| IBIS file stm32u595_599_5a5_5a9_lqfp144.ibs
[IBIS ver] 4.2
[File name] stm32u595_599_5a5_5a9_lqfp144.ibs
[File Rev] rev2.0
[Date]  11-09-2023
[Source] Data Created at STMicroelectronics
[Notes]  File originated from ELDO simulations.
[Disclaimer]  This information is for modeling purpose only and is
   not guaranteed. The information is subject to change without
   notice.
[Copyright] Copyright 2023 STMicroelectronics Inc.
|   Component stm32u595_599_5a5_5a9_lqfp144
[Component] stm32u595_599_5a5_5a9_lqfp144
[Manufacturer] STMicroelectronics
[Package]
| variable   typ   min   max
R_pkg  0  NA  NA
L_pkg  0  NA  NA
C_pkg  0  NA  NA
[Pin]   signal_name   model_name
1  PE2  io8_100m_hslv_ft
2  PE3  io8_100m_hslv_tamp_ft
3  PE4  io8_100m_hslv_tamp_ft
4  PE5  io8_100m_hslv_tamp_ft
5  PE6  io8_100m_hslv_tamp_ft
6  VBAT  power
7  PC13  io8_100m_ft
8  PC14-OSC32_IN  nc
9  PC15-OSC32_OUT  nc
10  PF0  io8_100m_hslv_ft
11  PF1  io8_100m_hslv_ft
12  PF2  io8_100m_hslv_ft
13  PF3  io8_100m_hslv_ft
14  PF4  io8_spi_ft
15  PF5  io8_spi_ft
16  VSS  gnd
17  VDD  power
18  PF6  io8_100m_hslv_ft
19  PF7  io8_100m_hslv_ft
20  PF8  io8_100m_hslv_ft
21  PF9  io8_100m_hslv_ft
22  PF10  io8_166m_hslv_ft
23  PH0-OSC_IN  nc
24  PH1-OSC_OUT   nc
25  NRST  nc
26  PC0  io8_100m_hslv_ft
27  PC1  io8_spi_hslv_ft
28  PC2  io8_100m_hslv_ft
29  PC3  io8_100m_hslv_ft
30  VSSA  nc
31  VREFM  nc
32  VREFP  nc
33  VDDA  nc
34  PA0  io8_100m_hslv_tamp_ft
35  PA1  io8_100m_hslv_tamp_ft
36  PA2  io8_100m_hslv_ft
37  PA3  io8_166m_hslv_ft
38  VSS  gnd
39  VDD  power
40  PA4  io8_100m_hslv_ft
41  PA5  io8_100m_ft
42  PA6  io8_100m_hslv_ft
43  PA7  io8_100m_hslv_ft
44  PC4  io8_100m_hslv_ft
45  PC5  io8_100m_tamp_ft
46  PB0  io8_100m_hslv_ft
47  PB1  io8_100m_hslv_ft
48  PB2  io8_100m_hslv_tamp_ft
49  PF11  io8_166m_hslv_ft
50  PF12  io8_100m_hslv_ft
51  VSS  gnd
52  VDD  power
53  PF13  io8_100m_hslv_ft
54  PF14  io8_100m_hslv_ft
55  PF15  io8_100m_hslv_ft
56  PG0  io8_100m_hslv_ft
57  PG1  io8_100m_hslv_ft
58  PE7  io8_100m_hslv_ft
59  PE8  io8_100m_hslv_ft
60  PE9  io8_166m_hslv_ft
61  VSS  gnd
62  VDD  power
63  PE10  io8_166m_hslv_ft
64  PE11  io8_100m_hslv_ft
65  PE12  io8_100m_hslv_ft
66  PE13  io8_100m_hslv_ft
67  PE14  io8_100m_hslv_ft
68  PE15  io8_100m_hslv_ft
69  PB10  io8_spi_hslv_ft
70  VCAP  nc
71  VSSA  nc
72  VDD  power
73  PB12  io8_166m_hslv_ft
74  PB13  io8_100m_i2c_ft
75  PB14  io8_100m_i2c_ft
76  PB15  nc
77  PD8  io8_100m_hslv_ft
78  PD9  io8_100m_hslv_ft
79  PD10  io8_100m_hslv_ft
80  PD11  io8_100m_hslv_ft
81  PD12  io8_100m_hslv_ft
82  PD13  io8_100m_hslv_ft
83  VSS  gnd
84  VDD  power
85  PD14  io8_100m_hslv_ft
86  PD15  io8_100m_hslv_ft
87  PG2  io8_100m_hslv_ft
88  PG3  io8_100m_hslv_ft
89  PG4  io8_100m_hslv_ft
90  PG5  io8_100m_hslv_ft
91  PG6  io8_100m_hslv_ft
92  PG7  io8_100m_hslv_ft
93  PG8  io8_100m_i2c_ft
94  VSS  gnd
95  VDDIO2  power
96  PC6  io8_100m_ft
97  PC7  io8_100m_ft
98  PC8  io8_100m_ft
99  PC9  io8_100m_ft
100  PA8  io8_166m_hslv_ft
101  PA9  io8_100m_usb_vbus_ft
102  PA10  io8_100m_usb_id
103  PA11  io8_100m_ft
104  PA12  io8_100m_ft
105  PA13  io8_100m_ft
106  VDDUSB  power
107  VSS  gnd
108  VDD  power
109  PA14  io8_100m_ft
110  PA15  nc
111  PC10  io8_100m_ft
112  PC11  io8_100m_hslv_ft
113  PC12  io8_166m_hslv_ft
114  PD0  io8_100m_hslv_ft
115  PD1  io8_100m_hslv_ft
116  PD2  io8_100m_ft
117  PD3  io8_166m_hslv_ft
118  PD4  io8_100m_hslv_ft
119  PD5  io8_100m_hslv_ft
120  VSS  gnd
121  VDD  power
122  PD6  io8_166m_hslv_ft
123  PD7  io8_100m_hslv_ft
124  PG9  io8_100m_hslv_ft
125  PG10  io8_100m_hslv_ft
126  PG11  io8_100m_hslv_ft
127  PG12  io8_100m_hslv_ft
128  PG13  io8_100m_hslv_ft
129  PG14  io8_100m_hslv_ft
130  VSS  gnd
131  VDDIO2  power
132  PG15  io8_100m_hslv_ft
133  PB3  io8_100m_i2c_ft
134  PB4  io8_100m_i2c_ft
135  PB5  io8_166m_hslv_ft
136  PB6  io8_100m_i2c_ft
137  PB7  io8_spi_hslv_ft
138  PH3-BOOT0  nc
139  PB8  io8_100m_i2c_ft
140  PB9  io8_100m_i2c_ft
141  PE0  io8_100m_hslv_ft
142  PE1  io8_100m_hslv_ft
143  VSS  gnd
144  VDD  power
[Package Model]   481-lqfp-20x20-144-ldo-230228
[Pin Mapping]   pulldown_ref   pullup_ref   | Comment
1  gndio  vddiom
2  gndio  vddiom
3  gndio  vddiom
4  gndio  vddiom
5  gndio  vddiom
6  nc  vsw
7  gndio  vddiom  | Depending on IO usage
| 7  gndio  vsw  | Depending on IO usage
8  nc  nc
9  nc  nc
10  gndio  vddiom
11  gndio  vddiom
12  gndio  vddiom
13  gndio  vddiom
14  gndio  vddiom
15  gndio  vddiom
16  gndio  nc
17  nc  vddiom
18  gndio  vddiom
19  gndio  vddiom
20  gndio  vddiom
21  gndio  vddiom
22  gndio  vddiom
23  nc  nc
24  nc  nc
25  nc  nc
26  gndio  vddiom
27  gndio  vddiom
28  gndio  vddiom
29  gndio  vddiom
30  nc  nc
31  nc  nc
32  nc  nc
33  nc  nc
34  gndio  vddiom
35  gndio  vddiom
36  gndio  vddiom
37  gndio  vddiom
38  gndio  nc
39  nc  vddiom
40  gndio  vddiom
41  gndio  vddiom
42  gndio  vddiom
43  gndio  vddiom
44  gndio  vddiom
45  gndio  vddiom
46  gndio  vddiom
47  gndio  vddiom
48  gndio  vddiom
49  gndio  vddiom
50  gndio  vddiom
51  gndio  nc
52  nc  vddiom
53  gndio  vddiom
54  gndio  vddiom
55  gndio  vddiom
56  gndio  vddiom
57  gndio  vddiom
58  gndio  vddiom
59  gndio  vddiom
60  gndio  vddiom
61  gndio  nc
62  nc  vddiom
63  gndio  vddiom
64  gndio  vddiom
65  gndio  vddiom
66  gndio  vddiom
67  gndio  vddiom
68  gndio  vddiom
69  gndio  vddiom
70  nc  nc
71  nc  nc
72  nc  vddiom
73  gndio  vddiom
74  gndio  vddiom
75  gndio  vddiom
76  nc  nc
77  gndio  vddiom
78  gndio  vddiom
79  gndio  vddiom
80  gndio  vddiom
81  gndio  vddiom
82  gndio  vddiom
83  gndio  nc
84  nc  vddiom
85  gndio  vddiom
86  gndio  vddiom
87  gndio  vddiom  | Depending on IO usage
| 87  gndio  vddio2  | Depending on IO usage
88  gndio  vddiom  | Depending on IO usage
| 88  gndio  vddio2  | Depending on IO usage
89  gndio  vddiom  | Depending on IO usage
| 89  gndio  vddio2  | Depending on IO usage
90  gndio  vddiom  | Depending on IO usage
| 90  gndio  vddio2  | Depending on IO usage
91  gndio  vddiom  | Depending on IO usage
| 91  gndio  vddio2  | Depending on IO usage
92  gndio  vddiom  | Depending on IO usage
| 92  gndio  vddio2  | Depending on IO usage
93  gndio  vddiom  | Depending on IO usage
| 93  gndio  vddio2  | Depending on IO usage
94  gndio  nc
95  nc  vddio2
96  gndio  vddiom
97  gndio  vddiom
98  gndio  vddiom
99  gndio  vddiom
100  gndio  vddiom
101  gndio  vddiom  | Depending on IO usage
| 101  gndio  vddusb  | Depending on IO usage
102  gndio  vddiom  | Depending on IO usage
| 102  gndio  vddusb  | Depending on IO usage
103  gndio  vddiom  | Depending on IO usage
| 103  gndio  vddusb  | Depending on IO usage
104  gndio  vddiom  | Depending on IO usage
| 104  gndio  vddusb  | Depending on IO usage
105  gndio  vddiom  | Depending on IO usage
| 105  gndio  vddusb  | Depending on IO usage
106  nc  vddusb
107  gndio  nc
108  nc  vddiom
109  gndio  vddiom
110  nc  nc
111  gndio  vddiom
112  gndio  vddiom
113  gndio  vddiom
114  gndio  vddiom
115  gndio  vddiom
116  gndio  vddiom
117  gndio  vddiom
118  gndio  vddiom
119  gndio  vddiom
120  gndio  nc
121  nc  vddiom
122  gndio  vddiom
123  gndio  vddiom
124  gndio  vddiom  | Depending on IO usage
| 124  gndio  vddio2  | Depending on IO usage
125  gndio  vddiom  | Depending on IO usage
| 125  gndio  vddio2  | Depending on IO usage
126  gndio  vddiom  | Depending on IO usage
| 126  gndio  vddio2  | Depending on IO usage
127  gndio  vddiom  | Depending on IO usage
| 127  gndio  vddio2  | Depending on IO usage
128  gndio  vddiom  | Depending on IO usage
| 128  gndio  vddio2  | Depending on IO usage
129  gndio  vddiom  | Depending on IO usage
| 129  gndio  vddio2  | Depending on IO usage
130  gndio  nc
131  nc  vddio2
132  gndio  vddiom  | Depending on IO usage
| 132  gndio  vddio2  | Depending on IO usage
133  gndio  vddiom
134  gndio  vddiom
135  gndio  vddiom
136  gndio  vddiom
137  gndio  vddiom
138  nc  nc
139  gndio  vddiom
140  gndio  vddiom
141  gndio  vddiom
142  gndio  vddiom
143  gndio  nc
144  nc  vddiom
[Model Selector] io8_100m_ft
io8_100m_ft_hs_1v2  "IO8_FT 100MHz high speed @ 1.2V"
io8_100m_ft_fs_1v2  "IO8_FT 100MHz fast speed @ 1.2V"
io8_100m_ft_fs_pd_1v2  "IO8_FT 100MHz fast speed @ 1.2V pulldown"
io8_100m_ft_ms_1v2  "IO8_FT 100MHz med speed @ 1.2V"
io8_100m_ft_ms_pd_1v2  "IO8_FT 100MHz med speed @ 1.2V pulldown"
io8_100m_ft_ls_1v2  "IO8_FT 100MHz low speed @ 1.2V"
io8_100m_ft_ls_pd_1v2  "IO8_FT 100MHz low speed @ 1.2V pulldown"
io8_100m_ft_hs_1v8  "IO8_FT 100MHz high speed @ 1.8V"
io8_100m_ft_hs_pd_1v8  "IO8_FT 100MHz high speed @ 1.8V pulldown"
io8_100m_ft_fs_1v8  "IO8_FT 100MHz fast speed @ 1.8V"
io8_100m_ft_fs_pd_1v8  "IO8_FT 100MHz fast speed @ 1.8V pulldown"
io8_100m_ft_ms_1v8  "IO8_FT 100MHz med speed @ 1.8V"
io8_100m_ft_ms_pd_1v8  "IO8_FT 100MHz med speed @ 1.8V pulldown"
io8_100m_ft_ls_1v8  "IO8_FT 100MHz low speed @ 1.8V"
io8_100m_ft_ls_pd_1v8  "IO8_FT 100MHz low speed @ 1.8V pulldown"
io8_100m_ft_hs_3v3  "IO8_FT 100MHz high speed @ 3.3V"
io8_100m_ft_hs_pd_3v3  "IO8_FT 100MHz high speed @ 3.3V pulldown"
io8_100m_ft_fs_3v3  "IO8_FT 100MHz fast speed @ 3.3V"
io8_100m_ft_fs_pd_3v3  "IO8_FT 100MHz fast speed @ 3.3V pulldown"
io8_100m_ft_ms_3v3  "IO8_FT 100MHz med speed @ 3.3V"
io8_100m_ft_ms_pd_3v3  "IO8_FT 100MHz med speed @ 3.3V pulldown"
io8_100m_ft_ls_3v3  "IO8_FT 100MHz low speed @ 3.3V"
io8_100m_ft_ls_pd_3v3  "IO8_FT 100MHz low speed @ 3.3V pulldown"
[Model Selector] io8_100m_hslv_ft
io8_100m_ft_hs_1v2  "IO8_FT 100MHz high speed @ 1.2V"
io8_100m_ft_hs_pu_1v2  "IO8_FT 100MHz high speed @ 1.2V pullup"
io8_100m_ft_hs_pd_1v2  "IO8_FT 100MHz high speed @ 1.2V pulldown"
io8_100m_ft_fs_1v2  "IO8_FT 100MHz fast speed @ 1.2V"
io8_100m_ft_fs_pu_1v2  "IO8_FT 100MHz fast speed @ 1.2V pullup"
io8_100m_ft_fs_pd_1v2  "IO8_FT 100MHz fast speed @ 1.2V pulldown"
io8_100m_ft_ms_1v2  "IO8_FT 100MHz med speed @ 1.2V"
io8_100m_ft_ms_pu_1v2  "IO8_FT 100MHz med speed @ 1.2V pullup"
io8_100m_ft_ms_pd_1v2  "IO8_FT 100MHz med speed @ 1.2V pulldown"
io8_100m_ft_ls_1v2  "IO8_FT 100MHz low speed @ 1.2V"
io8_100m_ft_ls_pu_1v2  "IO8_FT 100MHz low speed @ 1.2V pullup"
io8_100m_ft_ls_pd_1v2  "IO8_FT 100MHz low speed @ 1.2V pulldown"
io8_100m_ft_hs_1v8  "IO8_FT 100MHz high speed @ 1.8V"
io8_100m_ft_hs_pu_1v8  "IO8_FT 100MHz high speed @ 1.8V pullup"
io8_100m_ft_hs_pd_1v8  "IO8_FT 100MHz high speed @ 1.8V pulldown"
io8_100m_ft_fs_1v8  "IO8_FT 100MHz fast speed @ 1.8V"
io8_100m_ft_fs_pu_1v8  "IO8_FT 100MHz fast speed @ 1.8V pullup"
io8_100m_ft_fs_pd_1v8  "IO8_FT 100MHz fast speed @ 1.8V pulldown"
io8_100m_ft_ms_1v8  "IO8_FT 100MHz med speed @ 1.8V"
io8_100m_ft_ms_pu_1v8  "IO8_FT 100MHz med speed @ 1.8V pullup"
io8_100m_ft_ms_pd_1v8  "IO8_FT 100MHz med speed @ 1.8V pulldown"
io8_100m_ft_ls_1v8  "IO8_FT 100MHz low speed @ 1.8V"
io8_100m_ft_ls_pu_1v8  "IO8_FT 100MHz low speed @ 1.8V pullup"
io8_100m_ft_ls_pd_1v8  "IO8_FT 100MHz low speed @ 1.8V pulldown"
io8_100m_ft_hs_3v3  "IO8_FT 100MHz high speed @ 3.3V"
io8_100m_ft_hs_pu_3v3  "IO8_FT 100MHz high speed @ 3.3V pullup"
io8_100m_ft_hs_pd_3v3  "IO8_FT 100MHz high speed @ 3.3V pulldown"
io8_100m_ft_fs_3v3  "IO8_FT 100MHz fast speed @ 3.3V"
io8_100m_ft_fs_pu_3v3  "IO8_FT 100MHz fast speed @ 3.3V pullup"
io8_100m_ft_fs_pd_3v3  "IO8_FT 100MHz fast speed @ 3.3V pulldown"
io8_100m_ft_ms_3v3  "IO8_FT 100MHz med speed @ 3.3V"
io8_100m_ft_ms_pu_3v3  "IO8_FT 100MHz med speed @ 3.3V pullup"
io8_100m_ft_ms_pd_3v3  "IO8_FT 100MHz med speed @ 3.3V pulldown"
io8_100m_ft_ls_3v3  "IO8_FT 100MHz low speed @ 3.3V"
io8_100m_ft_ls_pu_3v3  "IO8_FT 100MHz low speed @ 3.3V pullup"
io8_100m_ft_ls_pd_3v3  "IO8_FT 100MHz low speed @ 3.3V pulldown"
io8_100m_hslv_ft_hs_1v2  "IO8_FT 100MHz HSLV high speed @ 1.2V"
io8_100m_hslv_ft_hs_pu_1v2  "IO8_FT 100MHz HSLV high speed @ 1.2V pullup"
io8_100m_hslv_ft_hs_pd_1v2  "IO8_FT 100MHz HSLV high speed @ 1.2V pulldown"
io8_100m_hslv_ft_fs_1v2  "IO8_FT 100MHz HSLV fast speed @ 1.2V"
io8_100m_hslv_ft_fs_pu_1v2  "IO8_FT 100MHz HSLV fast speed @ 1.2V pullup"
io8_100m_hslv_ft_fs_pd_1v2  "IO8_FT 100MHz HSLV fast speed @ 1.2V pulldown"
io8_100m_hslv_ft_ms_1v2  "IO8_FT 100MHz HSLV med speed @ 1.2V"
io8_100m_hslv_ft_ms_pu_1v2  "IO8_FT 100MHz HSLV med speed @ 1.2V pullup"
io8_100m_hslv_ft_ms_pd_1v2  "IO8_FT 100MHz HSLV med speed @ 1.2V pulldown"
io8_100m_hslv_ft_ls_1v2  "IO8_FT 100MHz HSLV low speed @ 1.2V"
io8_100m_hslv_ft_ls_pu_1v2  "IO8_FT 100MHz HSLV low speed @ 1.2V pullup"
io8_100m_hslv_ft_ls_pd_1v2  "IO8_FT 100MHz HSLV low speed @ 1.2V pulldown"
io8_100m_hslv_ft_hs_1v8  "IO8_FT 100MHz HSLV high speed @ 1.8V"
io8_100m_hslv_ft_hs_pu_1v8  "IO8_FT 100MHz HSLV high speed @ 1.8V pullup"
io8_100m_hslv_ft_hs_pd_1v8  "IO8_FT 100MHz HSLV high speed @ 1.8V pulldown"
io8_100m_hslv_ft_fs_1v8  "IO8_FT 100MHz HSLV fast speed @ 1.8V"
io8_100m_hslv_ft_fs_pu_1v8  "IO8_FT 100MHz HSLV fast speed @ 1.8V pullup"
io8_100m_hslv_ft_fs_pd_1v8  "IO8_FT 100MHz HSLV fast speed @ 1.8V pulldown"
io8_100m_hslv_ft_ms_1v8  "IO8_FT 100MHz HSLV med speed @ 1.8V"
io8_100m_hslv_ft_ms_pu_1v8  "IO8_FT 100MHz HSLV med speed @ 1.8V pullup"
io8_100m_hslv_ft_ms_pd_1v8  "IO8_FT 100MHz HSLV med speed @ 1.8V pulldown"
io8_100m_hslv_ft_ls_1v8  "IO8_FT 100MHz HSLV low speed @ 1.8V"
io8_100m_hslv_ft_ls_pu_1v8  "IO8_FT 100MHz HSLV low speed @ 1.8V pullup"
io8_100m_hslv_ft_ls_pd_1v8  "IO8_FT 100MHz HSLV low speed @ 1.8V pulldown"
io8_100m_hslv_ft_hs_2v5  "IO8_FT 100MHz HSLV high speed @ 2.5V"
io8_100m_hslv_ft_hs_pu_2v5  "IO8_FT 100MHz HSLV high speed @ 2.5V pullup"
io8_100m_hslv_ft_hs_pd_2v5  "IO8_FT 100MHz HSLV high speed @ 2.5V pulldown"
io8_100m_hslv_ft_fs_2v5  "IO8_FT 100MHz HSLV fast speed @ 2.5V"
io8_100m_hslv_ft_fs_pu_2v5  "IO8_FT 100MHz HSLV fast speed @ 2.5V pullup"
io8_100m_hslv_ft_fs_pd_2v5  "IO8_FT 100MHz HSLV fast speed @ 2.5V pulldown"
io8_100m_hslv_ft_ms_2v5  "IO8_FT 100MHz HSLV med speed @ 2.5V"
io8_100m_hslv_ft_ms_pu_2v5  "IO8_FT 100MHz HSLV med speed @ 2.5V pullup"
io8_100m_hslv_ft_ms_pd_2v5  "IO8_FT 100MHz HSLV med speed @ 2.5V pulldown"
io8_100m_hslv_ft_ls_2v5  "IO8_FT 100MHz HSLV low speed @ 2.5V"
io8_100m_hslv_ft_ls_pu_2v5  "IO8_FT 100MHz HSLV low speed @ 2.5V pullup"
io8_100m_hslv_ft_ls_pd_2v5  "IO8_FT 100MHz HSLV low speed @ 2.5V pulldown"
[Model Selector] io8_100m_hslv_tamp_ft
io8_100m_ft_hs_1v2  "IO8_FT 100MHz high speed @ 1.2V"
io8_100m_ft_hs_pu_1v2  "IO8_FT 100MHz high speed @ 1.2V pullup"
io8_100m_ft_hs_pd_1v2  "IO8_FT 100MHz high speed @ 1.2V pulldown"
io8_100m_ft_fs_1v2  "IO8_FT 100MHz fast speed @ 1.2V"
io8_100m_ft_fs_pu_1v2  "IO8_FT 100MHz fast speed @ 1.2V pullup"
io8_100m_ft_fs_pd_1v2  "IO8_FT 100MHz fast speed @ 1.2V pulldown"
io8_100m_ft_ms_1v2  "IO8_FT 100MHz med speed @ 1.2V"
io8_100m_ft_ms_pu_1v2  "IO8_FT 100MHz med speed @ 1.2V pullup"
io8_100m_ft_ms_pd_1v2  "IO8_FT 100MHz med speed @ 1.2V pulldown"
io8_100m_ft_ls_1v2  "IO8_FT 100MHz low speed @ 1.2V"
io8_100m_ft_ls_pu_1v2  "IO8_FT 100MHz low speed @ 1.2V pullup"
io8_100m_ft_ls_pd_1v2  "IO8_FT 100MHz low speed @ 1.2V pulldown"
io8_100m_ft_hs_1v8  "IO8_FT 100MHz high speed @ 1.8V"
io8_100m_ft_hs_pu_1v8  "IO8_FT 100MHz high speed @ 1.8V pullup"
io8_100m_ft_hs_pd_1v8  "IO8_FT 100MHz high speed @ 1.8V pulldown"
io8_100m_ft_fs_1v8  "IO8_FT 100MHz fast speed @ 1.8V"
io8_100m_ft_fs_pu_1v8  "IO8_FT 100MHz fast speed @ 1.8V pullup"
io8_100m_ft_fs_pd_1v8  "IO8_FT 100MHz fast speed @ 1.8V pulldown"
io8_100m_ft_ms_1v8  "IO8_FT 100MHz med speed @ 1.8V"
io8_100m_ft_ms_pu_1v8  "IO8_FT 100MHz med speed @ 1.8V pullup"
io8_100m_ft_ms_pd_1v8  "IO8_FT 100MHz med speed @ 1.8V pulldown"
io8_100m_ft_ls_1v8  "IO8_FT 100MHz low speed @ 1.8V"
io8_100m_ft_ls_pu_1v8  "IO8_FT 100MHz low speed @ 1.8V pullup"
io8_100m_ft_ls_pd_1v8  "IO8_FT 100MHz low speed @ 1.8V pulldown"
io8_100m_ft_hs_3v3  "IO8_FT 100MHz high speed @ 3.3V"
io8_100m_ft_hs_pu_3v3  "IO8_FT 100MHz high speed @ 3.3V pullup"
io8_100m_ft_hs_pd_3v3  "IO8_FT 100MHz high speed @ 3.3V pulldown"
io8_100m_ft_fs_3v3  "IO8_FT 100MHz fast speed @ 3.3V"
io8_100m_ft_fs_pu_3v3  "IO8_FT 100MHz fast speed @ 3.3V pullup"
io8_100m_ft_fs_pd_3v3  "IO8_FT 100MHz fast speed @ 3.3V pulldown"
io8_100m_ft_ms_3v3  "IO8_FT 100MHz med speed @ 3.3V"
io8_100m_ft_ms_pu_3v3  "IO8_FT 100MHz med speed @ 3.3V pullup"
io8_100m_ft_ms_pd_3v3  "IO8_FT 100MHz med speed @ 3.3V pulldown"
io8_100m_ft_ls_3v3  "IO8_FT 100MHz low speed @ 3.3V"
io8_100m_ft_ls_pu_3v3  "IO8_FT 100MHz low speed @ 3.3V pullup"
io8_100m_ft_ls_pd_3v3  "IO8_FT 100MHz low speed @ 3.3V pulldown"
io8_100m_hslv_ft_hs_1v2  "IO8_FT 100MHz HSLV high speed @ 1.2V"
io8_100m_hslv_ft_hs_pu_1v2  "IO8_FT 100MHz HSLV high speed @ 1.2V pullup"
io8_100m_hslv_ft_hs_pd_1v2  "IO8_FT 100MHz HSLV high speed @ 1.2V pulldown"
io8_100m_hslv_ft_fs_1v2  "IO8_FT 100MHz HSLV fast speed @ 1.2V"
io8_100m_hslv_ft_fs_pu_1v2  "IO8_FT 100MHz HSLV fast speed @ 1.2V pullup"
io8_100m_hslv_ft_fs_pd_1v2  "IO8_FT 100MHz HSLV fast speed @ 1.2V pulldown"
io8_100m_hslv_ft_ms_1v2  "IO8_FT 100MHz HSLV med speed @ 1.2V"
io8_100m_hslv_ft_ms_pu_1v2  "IO8_FT 100MHz HSLV med speed @ 1.2V pullup"
io8_100m_hslv_ft_ms_pd_1v2  "IO8_FT 100MHz HSLV med speed @ 1.2V pulldown"
io8_100m_hslv_ft_ls_1v2  "IO8_FT 100MHz HSLV low speed @ 1.2V"
io8_100m_hslv_ft_ls_pu_1v2  "IO8_FT 100MHz HSLV low speed @ 1.2V pullup"
io8_100m_hslv_ft_ls_pd_1v2  "IO8_FT 100MHz HSLV low speed @ 1.2V pulldown"
io8_100m_hslv_ft_hs_1v8  "IO8_FT 100MHz HSLV high speed @ 1.8V"
io8_100m_hslv_ft_hs_pu_1v8  "IO8_FT 100MHz HSLV high speed @ 1.8V pullup"
io8_100m_hslv_ft_hs_pd_1v8  "IO8_FT 100MHz HSLV high speed @ 1.8V pulldown"
io8_100m_hslv_ft_fs_1v8  "IO8_FT 100MHz HSLV fast speed @ 1.8V"
io8_100m_hslv_ft_fs_pu_1v8  "IO8_FT 100MHz HSLV fast speed @ 1.8V pullup"
io8_100m_hslv_ft_fs_pd_1v8  "IO8_FT 100MHz HSLV fast speed @ 1.8V pulldown"
io8_100m_hslv_ft_ms_1v8  "IO8_FT 100MHz HSLV med speed @ 1.8V"
io8_100m_hslv_ft_ms_pu_1v8  "IO8_FT 100MHz HSLV med speed @ 1.8V pullup"
io8_100m_hslv_ft_ms_pd_1v8  "IO8_FT 100MHz HSLV med speed @ 1.8V pulldown"
io8_100m_hslv_ft_ls_1v8  "IO8_FT 100MHz HSLV low speed @ 1.8V"
io8_100m_hslv_ft_ls_pu_1v8  "IO8_FT 100MHz HSLV low speed @ 1.8V pullup"
io8_100m_hslv_ft_ls_pd_1v8  "IO8_FT 100MHz HSLV low speed @ 1.8V pulldown"
io8_100m_hslv_ft_hs_2v5  "IO8_FT 100MHz HSLV high speed @ 2.5V"
io8_100m_hslv_ft_hs_pu_2v5  "IO8_FT 100MHz HSLV high speed @ 2.5V pullup"
io8_100m_hslv_ft_hs_pd_2v5  "IO8_FT 100MHz HSLV high speed @ 2.5V pulldown"
io8_100m_hslv_ft_fs_2v5  "IO8_FT 100MHz HSLV fast speed @ 2.5V"
io8_100m_hslv_ft_fs_pu_2v5  "IO8_FT 100MHz HSLV fast speed @ 2.5V pullup"
io8_100m_hslv_ft_fs_pd_2v5  "IO8_FT 100MHz HSLV fast speed @ 2.5V pulldown"
io8_100m_hslv_ft_ms_2v5  "IO8_FT 100MHz HSLV med speed @ 2.5V"
io8_100m_hslv_ft_ms_pu_2v5  "IO8_FT 100MHz HSLV med speed @ 2.5V pullup"
io8_100m_hslv_ft_ms_pd_2v5  "IO8_FT 100MHz HSLV med speed @ 2.5V pulldown"
io8_100m_hslv_ft_ls_2v5  "IO8_FT 100MHz HSLV low speed @ 2.5V"
io8_100m_hslv_ft_ls_pu_2v5  "IO8_FT 100MHz HSLV low speed @ 2.5V pullup"
io8_100m_hslv_ft_ls_pd_2v5  "IO8_FT 100MHz HSLV low speed @ 2.5V pulldown"
io8_ft_v33_hs_1v2  "IO8_FT_V33 high speed @ 1.2V"
io8_ft_v33_hs_pu_1v2  "IO8_FT_V33 high speed @ 1.2V pullup"
io8_ft_v33_hs_pd_1v2  "IO8_FT_V33 high speed @ 1.2V pulldown"
io8_ft_v33_fs_1v2  "IO8_FT_V33 fast speed @ 1.2V"
io8_ft_v33_fs_pu_1v2  "IO8_FT_V33 fast speed @ 1.2V pullup"
io8_ft_v33_fs_pd_1v2  "IO8_FT_V33 fast speed @ 1.2V pulldown"
io8_ft_v33_ms_1v2  "IO8_FT_V33 med speed @ 1.2V"
io8_ft_v33_ms_pu_1v2  "IO8_FT_V33 med speed @ 1.2V pullup"
io8_ft_v33_ms_pd_1v2  "IO8_FT_V33 med speed @ 1.2V pulldown"
io8_ft_v33_ls_1v2  "IO8_FT_V33 low speed @ 1.2V"
io8_ft_v33_ls_pu_1v2  "IO8_FT_V33 low speed @ 1.2V pullup"
io8_ft_v33_ls_pd_1v2  "IO8_FT_V33 low speed @ 1.2V pulldown"
io8_ft_v33_hs_1v8  "IO8_FT_V33 high speed @ 1.8V"
io8_ft_v33_hs_pu_1v8  "IO8_FT_V33 high speed @ 1.8V pullup"
io8_ft_v33_hs_pd_1v8  "IO8_FT_V33 high speed @ 1.8V pulldown"
io8_ft_v33_fs_1v8  "IO8_FT_V33 fast speed @ 1.8V"
io8_ft_v33_fs_pu_1v8  "IO8_FT_V33 fast speed @ 1.8V pullup"
io8_ft_v33_fs_pd_1v8  "IO8_FT_V33 fast speed @ 1.8V pulldown"
io8_ft_v33_ms_1v8  "IO8_FT_V33 med speed @ 1.8V"
io8_ft_v33_ms_pu_1v8  "IO8_FT_V33 med speed @ 1.8V pullup"
io8_ft_v33_ms_pd_1v8  "IO8_FT_V33 med speed @ 1.8V pulldown"
io8_ft_v33_ls_1v8  "IO8_FT_V33 low speed @ 1.8V"
io8_ft_v33_ls_pu_1v8  "IO8_FT_V33 low speed @ 1.8V pullup"
io8_ft_v33_ls_pd_1v8  "IO8_FT_V33 low speed @ 1.8V pulldown"
io8_ft_v33_hs_3v3  "IO8_FT_V33 high speed @ 3.3V"
io8_ft_v33_hs_pu_3v3  "IO8_FT_V33 high speed @ 3.3V pullup"
io8_ft_v33_hs_pd_3v3  "IO8_FT_V33 high speed @ 3.3V pulldown"
io8_ft_v33_fs_3v3  "IO8_FT_V33 fast speed @ 3.3V"
io8_ft_v33_fs_pu_3v3  "IO8_FT_V33 fast speed @ 3.3V pullup"
io8_ft_v33_fs_pd_3v3  "IO8_FT_V33 fast speed @ 3.3V pulldown"
io8_ft_v33_ms_3v3  "IO8_FT_V33 med speed @ 3.3V"
io8_ft_v33_ms_pu_3v3  "IO8_FT_V33 med speed @ 3.3V pullup"
io8_ft_v33_ms_pd_3v3  "IO8_FT_V33 med speed @ 3.3V pulldown"
io8_ft_v33_ls_3v3  "IO8_FT_V33 low speed @ 3.3V"
io8_ft_v33_ls_pu_3v3  "IO8_FT_V33 low speed @ 3.3V pullup"
io8_ft_v33_ls_pd_3v3  "IO8_FT_V33 low speed @ 3.3V pulldown"
[Model Selector] io8_100m_i2c_ft
io8_100m_ft_hs_1v2  "IO8_FT 100MHz high speed @ 1.2V"
io8_100m_ft_hs_pu_1v2  "IO8_FT 100MHz high speed @ 1.2V pullup"
io8_100m_ft_hs_pd_1v2  "IO8_FT 100MHz high speed @ 1.2V pulldown"
io8_100m_ft_fs_1v2  "IO8_FT 100MHz fast speed @ 1.2V"
io8_100m_ft_fs_pu_1v2  "IO8_FT 100MHz fast speed @ 1.2V pullup"
io8_100m_ft_fs_pd_1v2  "IO8_FT 100MHz fast speed @ 1.2V pulldown"
io8_100m_ft_ms_1v2  "IO8_FT 100MHz med speed @ 1.2V"
io8_100m_ft_ms_pu_1v2  "IO8_FT 100MHz med speed @ 1.2V pullup"
io8_100m_ft_ms_pd_1v2  "IO8_FT 100MHz med speed @ 1.2V pulldown"
io8_100m_ft_ls_1v2  "IO8_FT 100MHz low speed @ 1.2V"
io8_100m_ft_ls_pu_1v2  "IO8_FT 100MHz low speed @ 1.2V pullup"
io8_100m_ft_ls_pd_1v2  "IO8_FT 100MHz low speed @ 1.2V pulldown"
io8_100m_ft_hs_1v8  "IO8_FT 100MHz high speed @ 1.8V"
io8_100m_ft_hs_pu_1v8  "IO8_FT 100MHz high speed @ 1.8V pullup"
io8_100m_ft_hs_pd_1v8  "IO8_FT 100MHz high speed @ 1.8V pulldown"
io8_100m_ft_fs_1v8  "IO8_FT 100MHz fast speed @ 1.8V"
io8_100m_ft_fs_pu_1v8  "IO8_FT 100MHz fast speed @ 1.8V pullup"
io8_100m_ft_fs_pd_1v8  "IO8_FT 100MHz fast speed @ 1.8V pulldown"
io8_100m_ft_ms_1v8  "IO8_FT 100MHz med speed @ 1.8V"
io8_100m_ft_ms_pu_1v8  "IO8_FT 100MHz med speed @ 1.8V pullup"
io8_100m_ft_ms_pd_1v8  "IO8_FT 100MHz med speed @ 1.8V pulldown"
io8_100m_ft_ls_1v8  "IO8_FT 100MHz low speed @ 1.8V"
io8_100m_ft_ls_pu_1v8  "IO8_FT 100MHz low speed @ 1.8V pullup"
io8_100m_ft_ls_pd_1v8  "IO8_FT 100MHz low speed @ 1.8V pulldown"
io8_100m_ft_hs_3v3  "IO8_FT 100MHz high speed @ 3.3V"
io8_100m_ft_hs_pu_3v3  "IO8_FT 100MHz high speed @ 3.3V pullup"
io8_100m_ft_hs_pd_3v3  "IO8_FT 100MHz high speed @ 3.3V pulldown"
io8_100m_ft_fs_3v3  "IO8_FT 100MHz fast speed @ 3.3V"
io8_100m_ft_fs_pu_3v3  "IO8_FT 100MHz fast speed @ 3.3V pullup"
io8_100m_ft_fs_pd_3v3  "IO8_FT 100MHz fast speed @ 3.3V pulldown"
io8_100m_ft_ms_3v3  "IO8_FT 100MHz med speed @ 3.3V"
io8_100m_ft_ms_pu_3v3  "IO8_FT 100MHz med speed @ 3.3V pullup"
io8_100m_ft_ms_pd_3v3  "IO8_FT 100MHz med speed @ 3.3V pulldown"
io8_100m_ft_ls_3v3  "IO8_FT 100MHz low speed @ 3.3V"
io8_100m_ft_ls_pu_3v3  "IO8_FT 100MHz low speed @ 3.3V pullup"
io8_100m_ft_ls_pd_3v3  "IO8_FT 100MHz low speed @ 3.3V pulldown"
io8_100m_i2c_ft_1v2  "IO8_FT 100MHz I2C @ 1.2V"
io8_100m_i2c_ft_pu_1v2  "IO8_FT 100MHz I2C @ 1.2V pullup"
io8_100m_i2c_ft_pd_1v2  "IO8_FT 100MHz I2C @ 1.2V pulldown"
io8_100m_i2c_ft_1v8  "IO8_FT 100MHz I2C @ 1.8V"
io8_100m_i2c_ft_pu_1v8  "IO8_FT 100MHz I2C @ 1.8V pullup"
io8_100m_i2c_ft_pd_1v8  "IO8_FT 100MHz I2C @ 1,8V pulldown"
io8_100m_i2c_ft_3v3  "IO8_FT 100MHz I2C @ 3.3V"
io8_100m_i2c_ft_pu_3v3  "IO8_FT 100MHz I2C HSLV @ 3.3V pullup"
io8_100m_i2c_ft_pd_3v3  "IO8_FT 100MHz I2C @ 3.3V pulldown"
[Model Selector] io8_100m_tamp_ft
io8_100m_ft_hs_1v2  "IO8_FT 100MHz high speed @ 1.2V"
io8_100m_ft_hs_pu_1v2  "IO8_FT 100MHz high speed @ 1.2V pullup"
io8_100m_ft_hs_pd_1v2  "IO8_FT 100MHz high speed @ 1.2V pulldown"
io8_100m_ft_fs_1v2  "IO8_FT 100MHz fast speed @ 1.2V"
io8_100m_ft_fs_pu_1v2  "IO8_FT 100MHz fast speed @ 1.2V pullup"
io8_100m_ft_fs_pd_1v2  "IO8_FT 100MHz fast speed @ 1.2V pulldown"
io8_100m_ft_ms_1v2  "IO8_FT 100MHz med speed @ 1.2V"
io8_100m_ft_ms_pu_1v2  "IO8_FT 100MHz med speed @ 1.2V pullup"
io8_100m_ft_ms_pd_1v2  "IO8_FT 100MHz med speed @ 1.2V pulldown"
io8_100m_ft_ls_1v2  "IO8_FT 100MHz low speed @ 1.2V"
io8_100m_ft_ls_pu_1v2  "IO8_FT 100MHz low speed @ 1.2V pullup"
io8_100m_ft_ls_pd_1v2  "IO8_FT 100MHz low speed @ 1.2V pulldown"
io8_100m_ft_hs_1v8  "IO8_FT 100MHz high speed @ 1.8V"
io8_100m_ft_hs_pu_1v8  "IO8_FT 100MHz high speed @ 1.8V pullup"
io8_100m_ft_hs_pd_1v8  "IO8_FT 100MHz high speed @ 1.8V pulldown"
io8_100m_ft_fs_1v8  "IO8_FT 100MHz fast speed @ 1.8V"
io8_100m_ft_fs_pu_1v8  "IO8_FT 100MHz fast speed @ 1.8V pullup"
io8_100m_ft_fs_pd_1v8  "IO8_FT 100MHz fast speed @ 1.8V pulldown"
io8_100m_ft_ms_1v8  "IO8_FT 100MHz med speed @ 1.8V"
io8_100m_ft_ms_pu_1v8  "IO8_FT 100MHz med speed @ 1.8V pullup"
io8_100m_ft_ms_pd_1v8  "IO8_FT 100MHz med speed @ 1.8V pulldown"
io8_100m_ft_ls_1v8  "IO8_FT 100MHz low speed @ 1.8V"
io8_100m_ft_ls_pu_1v8  "IO8_FT 100MHz low speed @ 1.8V pullup"
io8_100m_ft_ls_pd_1v8  "IO8_FT 100MHz low speed @ 1.8V pulldown"
io8_100m_ft_hs_3v3  "IO8_FT 100MHz high speed @ 3.3V"
io8_100m_ft_hs_pu_3v3  "IO8_FT 100MHz high speed @ 3.3V pullup"
io8_100m_ft_hs_pd_3v3  "IO8_FT 100MHz high speed @ 3.3V pulldown"
io8_100m_ft_fs_3v3  "IO8_FT 100MHz fast speed @ 3.3V"
io8_100m_ft_fs_pu_3v3  "IO8_FT 100MHz fast speed @ 3.3V pullup"
io8_100m_ft_fs_pd_3v3  "IO8_FT 100MHz fast speed @ 3.3V pulldown"
io8_100m_ft_ms_3v3  "IO8_FT 100MHz med speed @ 3.3V"
io8_100m_ft_ms_pu_3v3  "IO8_FT 100MHz med speed @ 3.3V pullup"
io8_100m_ft_ms_pd_3v3  "IO8_FT 100MHz med speed @ 3.3V pulldown"
io8_100m_ft_ls_3v3  "IO8_FT 100MHz low speed @ 3.3V"
io8_100m_ft_ls_pu_3v3  "IO8_FT 100MHz low speed @ 3.3V pullup"
io8_100m_ft_ls_pd_3v3  "IO8_FT 100MHz low speed @ 3.3V pulldown"
io8_ft_v33_hs_1v2  "IO8_FT_V33 high speed @ 1.2V"
io8_ft_v33_hs_pu_1v2  "IO8_FT_V33 high speed @ 1.2V pullup"
io8_ft_v33_hs_pd_1v2  "IO8_FT_V33 high speed @ 1.2V pulldown"
io8_ft_v33_fs_1v2  "IO8_FT_V33 fast speed @ 1.2V"
io8_ft_v33_fs_pu_1v2  "IO8_FT_V33 fast speed @ 1.2V pullup"
io8_ft_v33_fs_pd_1v2  "IO8_FT_V33 fast speed @ 1.2V pulldown"
io8_ft_v33_ms_1v2  "IO8_FT_V33 med speed @ 1.2V"
io8_ft_v33_ms_pu_1v2  "IO8_FT_V33 med speed @ 1.2V pullup"
io8_ft_v33_ms_pd_1v2  "IO8_FT_V33 med speed @ 1.2V pulldown"
io8_ft_v33_ls_1v2  "IO8_FT_V33 low speed @ 1.2V"
io8_ft_v33_ls_pu_1v2  "IO8_FT_V33 low speed @ 1.2V pullup"
io8_ft_v33_ls_pd_1v2  "IO8_FT_V33 low speed @ 1.2V pulldown"
io8_ft_v33_hs_1v8  "IO8_FT_V33 high speed @ 1.8V"
io8_ft_v33_hs_pu_1v8  "IO8_FT_V33 high speed @ 1.8V pullup"
io8_ft_v33_hs_pd_1v8  "IO8_FT_V33 high speed @ 1.8V pulldown"
io8_ft_v33_fs_1v8  "IO8_FT_V33 fast speed @ 1.8V"
io8_ft_v33_fs_pu_1v8  "IO8_FT_V33 fast speed @ 1.8V pullup"
io8_ft_v33_fs_pd_1v8  "IO8_FT_V33 fast speed @ 1.8V pulldown"
io8_ft_v33_ms_1v8  "IO8_FT_V33 med speed @ 1.8V"
io8_ft_v33_ms_pu_1v8  "IO8_FT_V33 med speed @ 1.8V pullup"
io8_ft_v33_ms_pd_1v8  "IO8_FT_V33 med speed @ 1.8V pulldown"
io8_ft_v33_ls_1v8  "IO8_FT_V33 low speed @ 1.8V"
io8_ft_v33_ls_pu_1v8  "IO8_FT_V33 low speed @ 1.8V pullup"
io8_ft_v33_ls_pd_1v8  "IO8_FT_V33 low speed @ 1.8V pulldown"
io8_ft_v33_hs_3v3  "IO8_FT_V33 high speed @ 3.3V"
io8_ft_v33_hs_pu_3v3  "IO8_FT_V33 high speed @ 3.3V pullup"
io8_ft_v33_hs_pd_3v3  "IO8_FT_V33 high speed @ 3.3V pulldown"
io8_ft_v33_fs_3v3  "IO8_FT_V33 fast speed @ 3.3V"
io8_ft_v33_fs_pu_3v3  "IO8_FT_V33 fast speed @ 3.3V pullup"
io8_ft_v33_fs_pd_3v3  "IO8_FT_V33 fast speed @ 3.3V pulldown"
io8_ft_v33_ms_3v3  "IO8_FT_V33 med speed @ 3.3V"
io8_ft_v33_ms_pu_3v3  "IO8_FT_V33 med speed @ 3.3V pullup"
io8_ft_v33_ms_pd_3v3  "IO8_FT_V33 med speed @ 3.3V pulldown"
io8_ft_v33_ls_3v3  "IO8_FT_V33 low speed @ 3.3V"
io8_ft_v33_ls_pu_3v3  "IO8_FT_V33 low speed @ 3.3V pullup"
io8_ft_v33_ls_pd_3v3  "IO8_FT_V33 low speed @ 3.3V pulldown"
[Model Selector] io8_100m_usb_id
io8_100m_ft_hs_1v2  "IO8_FT 100MHz high speed @ 1.2V"
io8_100m_ft_hs_pu_1v2  "IO8_FT 100MHz high speed @ 1.2V pullup"
io8_100m_ft_hs_pd_1v2  "IO8_FT 100MHz high speed @ 1.2V pulldown"
io8_100m_ft_fs_1v2  "IO8_FT 100MHz fast speed @ 1.2V"
io8_100m_ft_fs_pu_1v2  "IO8_FT 100MHz fast speed @ 1.2V pullup"
io8_100m_ft_fs_pd_1v2  "IO8_FT 100MHz fast speed @ 1.2V pulldown"
io8_100m_ft_ms_1v2  "IO8_FT 100MHz med speed @ 1.2V"
io8_100m_ft_ms_pu_1v2  "IO8_FT 100MHz med speed @ 1.2V pullup"
io8_100m_ft_ms_pd_1v2  "IO8_FT 100MHz med speed @ 1.2V pulldown"
io8_100m_ft_ls_1v2  "IO8_FT 100MHz low speed @ 1.2V"
io8_100m_ft_ls_pu_1v2  "IO8_FT 100MHz low speed @ 1.2V pullup"
io8_100m_ft_ls_pd_1v2  "IO8_FT 100MHz low speed @ 1.2V pulldown"
io8_100m_ft_hs_1v8  "IO8_FT 100MHz high speed @ 1.8V"
io8_100m_ft_hs_pu_1v8  "IO8_FT 100MHz high speed @ 1.8V pullup"
io8_100m_ft_hs_pd_1v8  "IO8_FT 100MHz high speed @ 1.8V pulldown"
io8_100m_ft_fs_1v8  "IO8_FT 100MHz fast speed @ 1.8V"
io8_100m_ft_fs_pu_1v8  "IO8_FT 100MHz fast speed @ 1.8V pullup"
io8_100m_ft_fs_pd_1v8  "IO8_FT 100MHz fast speed @ 1.8V pulldown"
io8_100m_ft_ms_1v8  "IO8_FT 100MHz med speed @ 1.8V"
io8_100m_ft_ms_pu_1v8  "IO8_FT 100MHz med speed @ 1.8V pullup"
io8_100m_ft_ms_pd_1v8  "IO8_FT 100MHz med speed @ 1.8V pulldown"
io8_100m_ft_ls_1v8  "IO8_FT 100MHz low speed @ 1.8V"
io8_100m_ft_ls_pu_1v8  "IO8_FT 100MHz low speed @ 1.8V pullup"
io8_100m_ft_ls_pd_1v8  "IO8_FT 100MHz low speed @ 1.8V pulldown"
io8_100m_ft_hs_3v3  "IO8_FT 100MHz high speed @ 3.3V"
io8_100m_ft_hs_pu_3v3  "IO8_FT 100MHz high speed @ 3.3V pullup"
io8_100m_ft_hs_pd_3v3  "IO8_FT 100MHz high speed @ 3.3V pulldown"
io8_100m_ft_fs_3v3  "IO8_FT 100MHz fast speed @ 3.3V"
io8_100m_ft_fs_pu_3v3  "IO8_FT 100MHz fast speed @ 3.3V pullup"
io8_100m_ft_fs_pd_3v3  "IO8_FT 100MHz fast speed @ 3.3V pulldown"
io8_100m_ft_ms_3v3  "IO8_FT 100MHz med speed @ 3.3V"
io8_100m_ft_ms_pu_3v3  "IO8_FT 100MHz med speed @ 3.3V pullup"
io8_100m_ft_ms_pd_3v3  "IO8_FT 100MHz med speed @ 3.3V pulldown"
io8_100m_ft_ls_3v3  "IO8_FT 100MHz low speed @ 3.3V"
io8_100m_ft_ls_pu_3v3  "IO8_FT 100MHz low speed @ 3.3V pullup"
io8_100m_ft_ls_pd_3v3  "IO8_FT 100MHz low speed @ 3.3V pulldown"
io8usb_id_nopu  "IOUSB ID @ 3.3V"
io8usb_id_pu  "IOUSB ID @ 3.3V pullup"
[Model Selector] io8_100m_usb_vbus_ft
io8_100m_ft_hs_1v2  "IO8_FT 100MHz high speed @ 1.2V"
io8_100m_ft_hs_pu_1v2  "IO8_FT 100MHz high speed @ 1.2V pullup"
io8_100m_ft_hs_pd_1v2  "IO8_FT 100MHz high speed @ 1.2V pulldown"
io8_100m_ft_fs_1v2  "IO8_FT 100MHz fast speed @ 1.2V"
io8_100m_ft_fs_pu_1v2  "IO8_FT 100MHz fast speed @ 1.2V pullup"
io8_100m_ft_fs_pd_1v2  "IO8_FT 100MHz fast speed @ 1.2V pulldown"
io8_100m_ft_ms_1v2  "IO8_FT 100MHz med speed @ 1.2V"
io8_100m_ft_ms_pu_1v2  "IO8_FT 100MHz med speed @ 1.2V pullup"
io8_100m_ft_ms_pd_1v2  "IO8_FT 100MHz med speed @ 1.2V pulldown"
io8_100m_ft_ls_1v2  "IO8_FT 100MHz low speed @ 1.2V"
io8_100m_ft_ls_pu_1v2  "IO8_FT 100MHz low speed @ 1.2V pullup"
io8_100m_ft_ls_pd_1v2  "IO8_FT 100MHz low speed @ 1.2V pulldown"
io8_100m_ft_hs_1v8  "IO8_FT 100MHz high speed @ 1.8V"
io8_100m_ft_hs_pu_1v8  "IO8_FT 100MHz high speed @ 1.8V pullup"
io8_100m_ft_hs_pd_1v8  "IO8_FT 100MHz high speed @ 1.8V pulldown"
io8_100m_ft_fs_1v8  "IO8_FT 100MHz fast speed @ 1.8V"
io8_100m_ft_fs_pu_1v8  "IO8_FT 100MHz fast speed @ 1.8V pullup"
io8_100m_ft_fs_pd_1v8  "IO8_FT 100MHz fast speed @ 1.8V pulldown"
io8_100m_ft_ms_1v8  "IO8_FT 100MHz med speed @ 1.8V"
io8_100m_ft_ms_pu_1v8  "IO8_FT 100MHz med speed @ 1.8V pullup"
io8_100m_ft_ms_pd_1v8  "IO8_FT 100MHz med speed @ 1.8V pulldown"
io8_100m_ft_ls_1v8  "IO8_FT 100MHz low speed @ 1.8V"
io8_100m_ft_ls_pu_1v8  "IO8_FT 100MHz low speed @ 1.8V pullup"
io8_100m_ft_ls_pd_1v8  "IO8_FT 100MHz low speed @ 1.8V pulldown"
io8_100m_ft_hs_3v3  "IO8_FT 100MHz high speed @ 3.3V"
io8_100m_ft_hs_pu_3v3  "IO8_FT 100MHz high speed @ 3.3V pullup"
io8_100m_ft_hs_pd_3v3  "IO8_FT 100MHz high speed @ 3.3V pulldown"
io8_100m_ft_fs_3v3  "IO8_FT 100MHz fast speed @ 3.3V"
io8_100m_ft_fs_pu_3v3  "IO8_FT 100MHz fast speed @ 3.3V pullup"
io8_100m_ft_fs_pd_3v3  "IO8_FT 100MHz fast speed @ 3.3V pulldown"
io8_100m_ft_ms_3v3  "IO8_FT 100MHz med speed @ 3.3V"
io8_100m_ft_ms_pu_3v3  "IO8_FT 100MHz med speed @ 3.3V pullup"
io8_100m_ft_ms_pd_3v3  "IO8_FT 100MHz med speed @ 3.3V pulldown"
io8_100m_ft_ls_3v3  "IO8_FT 100MHz low speed @ 3.3V"
io8_100m_ft_ls_pu_3v3  "IO8_FT 100MHz low speed @ 3.3V pullup"
io8_100m_ft_ls_pd_3v3  "IO8_FT 100MHz low speed @ 3.3V pulldown"
io8usb_adp "IOUSB ADP @ 3.3V"
io8usb_vbus "IOUSB VBUS @ 3.3V"
[Model Selector] io8_166m_hslv_ft
io8_166m_ft_hs_1v2  "IO8_FT 166MHz high speed @ 1.2V"
io8_166m_ft_hs_pu_1v2  "IO8_FT 166MHz high speed @ 1.2V pullup"
io8_166m_ft_hs_pd_1v2  "IO8_FT 166MHz high speed @ 1.2V pulldown"
io8_166m_ft_fs_1v2  "IO8_FT 166MHz fast speed @ 1.2V"
io8_166m_ft_fs_pu_1v2  "IO8_FT 166MHz fast speed @ 1.2V pullup"
io8_166m_ft_fs_pd_1v2  "IO8_FT 166MHz fast speed @ 1.2V pulldown"
io8_166m_ft_ms_1v2  "IO8_FT 166MHz med speed @ 1.2V"
io8_166m_ft_ms_pu_1v2  "IO8_FT 166MHz med speed @ 1.2V pullup"
io8_166m_ft_ms_pd_1v2  "IO8_FT 166MHz med speed @ 1.2V pulldown"
io8_166m_ft_ls_1v2  "IO8_FT 166MHz low speed @ 1.2V"
io8_166m_ft_ls_pu_1v2  "IO8_FT 166MHz low speed @ 1.2V pullup"
io8_166m_ft_ls_pd_1v2  "IO8_FT 166MHz low speed @ 1.2V pulldown"
io8_166m_ft_hs_1v8  "IO8_FT 166MHz high speed @ 1.8V"
io8_166m_ft_hs_pu_1v8  "IO8_FT 166MHz high speed @ 1.8V pullup"
io8_166m_ft_hs_pd_1v8  "IO8_FT 166MHz high speed @ 1.8V pulldown"
io8_166m_ft_fs_1v8  "IO8_FT 166MHz fast speed @ 1.8V"
io8_166m_ft_fs_pu_1v8  "IO8_FT 166MHz fast speed @ 1.8V pullup"
io8_166m_ft_fs_pd_1v8  "IO8_FT 166MHz fast speed @ 1.8V pulldown"
io8_166m_ft_ms_1v8  "IO8_FT 166MHz med speed @ 1.8V"
io8_166m_ft_ms_pu_1v8  "IO8_FT 166MHz med speed @ 1.8V pullup"
io8_166m_ft_ms_pd_1v8  "IO8_FT 166MHz med speed @ 1.8V pulldown"
io8_166m_ft_ls_1v8  "IO8_FT 166MHz low speed @ 1.8V"
io8_166m_ft_ls_pu_1v8  "IO8_FT 166MHz low speed @ 1.8V pullup"
io8_166m_ft_ls_pd_1v8  "IO8_FT 166MHz low speed @ 1.8V pulldown"
io8_166m_ft_hs_3v3  "IO8_FT 166MHz high speed @ 3.3V"
io8_166m_ft_hs_pu_3v3  "IO8_FT 166MHz high speed @ 3.3V pullup"
io8_166m_ft_hs_pd_3v3  "IO8_FT 166MHz high speed @ 3.3V pulldown"
io8_166m_ft_fs_3v3  "IO8_FT 166MHz fast speed @ 3.3V"
io8_166m_ft_fs_pu_3v3  "IO8_FT 166MHz fast speed @ 3.3V pullup"
io8_166m_ft_fs_pd_3v3  "IO8_FT 166MHz fast speed @ 3.3V pulldown"
io8_166m_ft_ms_3v3  "IO8_FT 166MHz med speed @ 3.3V"
io8_166m_ft_ms_pu_3v3  "IO8_FT 166MHz med speed @ 3.3V pullup"
io8_166m_ft_ms_pd_3v3  "IO8_FT 166MHz med speed @ 3.3V pulldown"
io8_166m_ft_ls_3v3  "IO8_FT 166MHz low speed @ 3.3V"
io8_166m_ft_ls_pu_3v3  "IO8_FT 166MHz low speed @ 3.3V pullup"
io8_166m_ft_ls_pd_3v3  "IO8_FT 166MHz low speed @ 3.3V pulldown"
io8_166m_hslv_ft_hs_1v2  "IO8_FT 166MHz HSLV high speed @ 1.2V"
io8_166m_hslv_ft_hs_pu_1v2  "IO8_FT 166MHz HSLV high speed @ 1.2V pullup"
io8_166m_hslv_ft_hs_pd_1v2  "IO8_FT 166MHz HSLV high speed @ 1.2V pulldown"
io8_166m_hslv_ft_fs_1v2  "IO8_FT 166MHz HSLV fast speed @ 1.2V"
io8_166m_hslv_ft_fs_pu_1v2  "IO8_FT 166MHz HSLV fast speed @ 1.2V pullup"
io8_166m_hslv_ft_fs_pd_1v2  "IO8_FT 166MHz HSLV fast speed @ 1.2V pulldown"
io8_166m_hslv_ft_ms_1v2  "IO8_FT 166MHz HSLV med speed @ 1.2V"
io8_166m_hslv_ft_ms_pu_1v2  "IO8_FT 166MHz HSLV med speed @ 1.2V pullup"
io8_166m_hslv_ft_ms_pd_1v2  "IO8_FT 166MHz HSLV med speed @ 1.2V pulldown"
io8_166m_hslv_ft_ls_1v2  "IO8_FT 166MHz HSLV low speed @ 1.2V"
io8_166m_hslv_ft_ls_pu_1v2  "IO8_FT 166MHz HSLV low speed @ 1.2V pullup"
io8_166m_hslv_ft_ls_pd_1v2  "IO8_FT 166MHz HSLV low speed @ 1.2V pulldown"
io8_166m_hslv_ft_hs_1v8  "IO8_FT 166MHz HSLV high speed @ 1.8V"
io8_166m_hslv_ft_hs_pu_1v8  "IO8_FT 166MHz HSLV high speed @ 1.8V pullup"
io8_166m_hslv_ft_hs_pd_1v8  "IO8_FT 166MHz HSLV high speed @ 1.8V pulldown"
io8_166m_hslv_ft_fs_1v8  "IO8_FT 166MHz HSLV fast speed @ 1.8V"
io8_166m_hslv_ft_fs_pu_1v8  "IO8_FT 166MHz HSLV fast speed @ 1.8V pullup"
io8_166m_hslv_ft_fs_pd_1v8  "IO8_FT 166MHz HSLV fast speed @ 1.8V pulldown"
io8_166m_hslv_ft_ms_1v8  "IO8_FT 166MHz HSLV med speed @ 1.8V"
io8_166m_hslv_ft_ms_pu_1v8  "IO8_FT 166MHz HSLV med speed @ 1.8V pullup"
io8_166m_hslv_ft_ms_pd_1v8  "IO8_FT 166MHz HSLV med speed @ 1.8V pulldown"
io8_166m_hslv_ft_ls_1v8  "IO8_FT 166MHz HSLV low speed @ 1.8V"
io8_166m_hslv_ft_ls_pu_1v8  "IO8_FT 166MHz HSLV low speed @ 1.8V pullup"
io8_166m_hslv_ft_ls_pd_1v8  "IO8_FT 166MHz HSLV low speed @ 1.8V pulldown"
io8_166m_hslv_ft_hs_2v5  "IO8_FT 166MHz HSLV high speed @ 2.5V"
io8_166m_hslv_ft_hs_pu_2v5  "IO8_FT 166MHz HSLV high speed @ 2.5V pullup"
io8_166m_hslv_ft_hs_pd_2v5  "IO8_FT 166MHz HSLV high speed @ 2.5V pulldown"
io8_166m_hslv_ft_fs_2v5  "IO8_FT 166MHz HSLV fast speed @ 2.5V"
io8_166m_hslv_ft_fs_pu_2v5  "IO8_FT 166MHz HSLV fast speed @ 2.5V pullup"
io8_166m_hslv_ft_fs_pd_2v5  "IO8_FT 166MHz HSLV fast speed @ 2.5V pulldown"
io8_166m_hslv_ft_ms_2v5  "IO8_FT 166MHz HSLV med speed @ 2.5V"
io8_166m_hslv_ft_ms_pu_2v5  "IO8_FT 166MHz HSLV med speed @ 2.5V pullup"
io8_166m_hslv_ft_ms_pd_2v5  "IO8_FT 166MHz HSLV med speed @ 2.5V pulldown"
io8_166m_hslv_ft_ls_2v5  "IO8_FT 166MHz HSLV low speed @ 2.5V"
io8_166m_hslv_ft_ls_pu_2v5  "IO8_FT 166MHz HSLV low speed @ 2.5V pullup"
io8_166m_hslv_ft_ls_pd_2v5  "IO8_FT 166MHz HSLV low speed @ 2.5V pulldown"
[Model Selector] io8_spi_hslv_ft
io8_spi_ft_hs_1v2  "IO8_FT SPI high speed @ 1.2V"
io8_spi_ft_hs_pu_1v2  "IO8_FT SPI high speed @ 1.2V pullup"
io8_spi_ft_hs_pd_1v2  "IO8_FT SPI high speed @ 1.2V pulldown"
io8_spi_ft_fs_1v2  "IO8_FT SPI fast speed @ 1.2V"
io8_spi_ft_fs_pu_1v2  "IO8_FT SPI fast speed @ 1.2V pullup"
io8_spi_ft_fs_pd_1v2  "IO8_FT SPI fast speed @ 1.2V pulldown"
io8_spi_ft_ms_1v2  "IO8_FT SPI med speed @ 1.2V"
io8_spi_ft_ms_pu_1v2  "IO8_FT SPI med speed @ 1.2V pullup"
io8_spi_ft_ms_pd_1v2  "IO8_FT SPI med speed @ 1.2V pulldown"
io8_spi_ft_ls_1v2  "IO8_FT SPI low speed @ 1.2V"
io8_spi_ft_ls_pu_1v2  "IO8_FT SPI low speed @ 1.2V pullup"
io8_spi_ft_ls_pd_1v2  "IO8_FT SPI low speed @ 1.2V pulldown"
io8_spi_ft_hs_1v8  "IO8_FT SPI high speed @ 1.8V"
io8_spi_ft_hs_pu_1v8  "IO8_FT SPI high speed @ 1.8V pullup"
io8_spi_ft_hs_pd_1v8  "IO8_FT SPI high speed @ 1.8V pulldown"
io8_spi_ft_fs_1v8  "IO8_FT SPI fast speed @ 1.8V"
io8_spi_ft_fs_pu_1v8  "IO8_FT SPI fast speed @ 1.8V pullup"
io8_spi_ft_fs_pd_1v8  "IO8_FT SPI fast speed @ 1.8V pulldown"
io8_spi_ft_ms_1v8  "IO8_FT SPI med speed @ 1.8V"
io8_spi_ft_ms_pu_1v8  "IO8_FT SPI med speed @ 1.8V pullup"
io8_spi_ft_ms_pd_1v8  "IO8_FT SPI med speed @ 1.8V pulldown"
io8_spi_ft_ls_1v8  "IO8_FT SPI low speed @ 1.8V"
io8_spi_ft_ls_pu_1v8  "IO8_FT SPI low speed @ 1.8V pullup"
io8_spi_ft_ls_pd_1v8  "IO8_FT SPI low speed @ 1.8V pulldown"
io8_spi_ft_hs_3v3  "IO8_FT SPI high speed @ 3.3V"
io8_spi_ft_hs_pu_3v3  "IO8_FT SPI high speed @ 3.3V pullup"
io8_spi_ft_hs_pd_3v3  "IO8_FT SPI high speed @ 3.3V pulldown"
io8_spi_ft_fs_3v3  "IO8_FT SPI fast speed @ 3.3V"
io8_spi_ft_fs_pu_3v3  "IO8_FT SPI fast speed @ 3.3V pullup"
io8_spi_ft_fs_pd_3v3  "IO8_FT SPI fast speed @ 3.3V pulldown"
io8_spi_ft_ms_3v3  "IO8_FT SPI med speed @ 3.3V"
io8_spi_ft_ms_pu_3v3  "IO8_FT SPI med speed @ 1.8V pullup"
io8_spi_ft_ms_pd_3v3  "IO8_FT SPI med speed @ 3.3V pulldown"
io8_spi_ft_ls_3v3  "IO8_FT SPI low speed @ 3.3V"
io8_spi_ft_ls_pu_3v3  "IO8_FT SPI low speed @ 3.3V pullup"
io8_spi_ft_ls_pd_3v3  "IO8_FT SPI low speed @ 3.3V pulldown"
io8_spi_hslv_ft_hs_1v2  "IO8_FT SPI HSLV high speed @ 1.2V"
io8_spi_hslv_ft_hs_pu_1v2  "IO8_FT SPI HSLV high speed @ 1.2V pullup"
io8_spi_hslv_ft_hs_pd_1v2  "IO8_FT SPI HSLV high speed @ 1.2V pulldown"
io8_spi_hslv_ft_fs_1v2  "IO8_FT SPI HSLV fast speed @ 1.2V"
io8_spi_hslv_ft_fs_pu_1v2  "IO8_FT SPI HSLV fast speed @ 1.2V pullup"
io8_spi_hslv_ft_fs_pd_1v2  "IO8_FT SPI HSLV fast speed @ 1.2V pulldown"
io8_spi_hslv_ft_ms_1v2  "IO8_FT SPI HSLV med speed @ 1.2V"
io8_spi_hslv_ft_ms_pu_1v2  "IO8_FT SPI HSLV med speed @ 1.2V pullup"
io8_spi_hslv_ft_ms_pd_1v2  "IO8_FT SPI HSLV med speed @ 1.2V pulldown"
io8_spi_hslv_ft_ls_1v2  "IO8_FT SPI HSLV low speed @ 1.2V"
io8_spi_hslv_ft_ls_pu_1v2  "IO8_FT SPI HSLV low speed @ 1.2V pullup"
io8_spi_hslv_ft_ls_pd_1v2  "IO8_FT SPI HSLV low speed @ 1.2V pulldown"
io8_spi_hslv_ft_hs_1v8  "IO8_FT SPI HSLV high speed @ 1.8V"
io8_spi_hslv_ft_hs_pu_1v8  "IO8_FT SPI HSLV high speed @ 1.8V pullup"
io8_spi_hslv_ft_hs_pd_1v8  "IO8_FT SPI HSLV high speed @ 1.8V pulldown"
io8_spi_hslv_ft_fs_1v8  "IO8_FT SPI HSLV fast speed @ 1.8V"
io8_spi_hslv_ft_fs_pu_1v8  "IO8_FT SPI HSLV fast speed @ 1.8V pullup"
io8_spi_hslv_ft_fs_pd_1v8  "IO8_FT SPI HSLV fast speed @ 1.8V pulldown"
io8_spi_hslv_ft_ms_1v8  "IO8_FT SPI HSLV med speed @ 1.8V"
io8_spi_hslv_ft_ms_pu_1v8  "IO8_FT SPI HSLV med speed @ 1.8V pullup"
io8_spi_hslv_ft_ms_pd_1v8  "IO8_FT SPI HSLV med speed @ 1.8V pulldown"
io8_spi_hslv_ft_ls_1v8  "IO8_FT SPI HSLV low speed @ 1.8V"
io8_spi_hslv_ft_ls_pu_1v8  "IO8_FT SPI HSLV low speed @ 1.8V pullup"
io8_spi_hslv_ft_ls_pd_1v8  "IO8_FT SPI HSLV low speed @ 1.8V pulldown"
io8_spi_hslv_ft_hs_2v5  "IO8_FT SPI HSLV high speed @ 2.5V"
io8_spi_hslv_ft_hs_pu_2v5  "IO8_FT SPI HSLV high speed @ 2.5V pullup"
io8_spi_hslv_ft_hs_pd_2v5  "IO8_FT SPI HSLV high speed @ 2.5V pulldown"
io8_spi_hslv_ft_fs_2v5  "IO8_FT SPI HSLV fast speed @ 2.5V"
io8_spi_hslv_ft_fs_pu_2v5  "IO8_FT SPI HSLV fast speed @ 2.5V pullup"
io8_spi_hslv_ft_fs_pd_2v5  "IO8_FT SPI HSLV fast speed @ 2.5V pulldown"
io8_spi_hslv_ft_ms_2v5  "IO8_FT SPI HSLV med speed @ 2.5V"
io8_spi_hslv_ft_ms_pu_2v5  "IO8_FT SPI HSLV med speed @ 2.5V pullup"
io8_spi_hslv_ft_ms_pd_2v5  "IO8_FT SPI HSLV med speed @ 2.5V pulldown"
io8_spi_hslv_ft_ls_2v5  "IO8_FT SPI HSLV low speed @ 2.5V"
io8_spi_hslv_ft_ls_pu_2v5  "IO8_FT SPI HSLV low speed @ 2.5V pullup"
io8_spi_hslv_ft_ls_pd_2v5  "IO8_FT SPI HSLV low speed @ 2.5V pulldown"
[Model Selector] io8_spi_ft
io8_spi_ft_hs_1v2  "IO8_FT SPI high speed @ 1.2V"
io8_spi_ft_hs_pu_1v2  "IO8_FT SPI high speed @ 1.2V pullup"
io8_spi_ft_hs_pd_1v2  "IO8_FT SPI high speed @ 1.2V pulldown"
io8_spi_ft_fs_1v2  "IO8_FT SPI fast speed @ 1.2V"
io8_spi_ft_fs_pu_1v2  "IO8_FT SPI fast speed @ 1.2V pullup"
io8_spi_ft_fs_pd_1v2  "IO8_FT SPI fast speed @ 1.2V pulldown"
io8_spi_ft_ms_1v2  "IO8_FT SPI med speed @ 1.2V"
io8_spi_ft_ms_pu_1v2  "IO8_FT SPI med speed @ 1.2V pullup"
io8_spi_ft_ms_pd_1v2  "IO8_FT SPI med speed @ 1.2V pulldown"
io8_spi_ft_ls_1v2  "IO8_FT SPI low speed @ 1.2V"
io8_spi_ft_ls_pu_1v2  "IO8_FT SPI low speed @ 1.2V pullup"
io8_spi_ft_ls_pd_1v2  "IO8_FT SPI low speed @ 1.2V pulldown"
io8_spi_ft_hs_1v8  "IO8_FT SPI high speed @ 1.8V"
io8_spi_ft_hs_pu_1v8  "IO8_FT SPI high speed @ 1.8V pullup"
io8_spi_ft_hs_pd_1v8  "IO8_FT SPI high speed @ 1.8V pulldown"
io8_spi_ft_fs_1v8  "IO8_FT SPI fast speed @ 1.8V"
io8_spi_ft_fs_pu_1v8  "IO8_FT SPI fast speed @ 1.8V pullup"
io8_spi_ft_fs_pd_1v8  "IO8_FT SPI fast speed @ 1.8V pulldown"
io8_spi_ft_ms_1v8  "IO8_FT SPI med speed @ 1.8V"
io8_spi_ft_ms_pu_1v8  "IO8_FT SPI med speed @ 1.8V pullup"
io8_spi_ft_ms_pd_1v8  "IO8_FT SPI med speed @ 1.8V pulldown"
io8_spi_ft_ls_1v8  "IO8_FT SPI low speed @ 1.8V"
io8_spi_ft_ls_pu_1v8  "IO8_FT SPI low speed @ 1.8V pullup"
io8_spi_ft_ls_pd_1v8  "IO8_FT SPI low speed @ 1.8V pulldown"
io8_spi_ft_hs_3v3  "IO8_FT SPI high speed @ 3.3V"
io8_spi_ft_hs_pu_3v3  "IO8_FT SPI high speed @ 3.3V pullup"
io8_spi_ft_hs_pd_3v3  "IO8_FT SPI high speed @ 3.3V pulldown"
io8_spi_ft_fs_3v3  "IO8_FT SPI fast speed @ 3.3V"
io8_spi_ft_fs_pu_3v3  "IO8_FT SPI fast speed @ 3.3V pullup"
io8_spi_ft_fs_pd_3v3  "IO8_FT SPI fast speed @ 3.3V pulldown"
io8_spi_ft_ms_3v3  "IO8_FT SPI med speed @ 3.3V"
io8_spi_ft_ms_pu_3v3  "IO8_FT SPI med speed @ 1.8V pullup"
io8_spi_ft_ms_pd_3v3  "IO8_FT SPI med speed @ 3.3V pulldown"
io8_spi_ft_ls_3v3  "IO8_FT SPI low speed @ 3.3V"
io8_spi_ft_ls_pu_3v3  "IO8_FT SPI low speed @ 3.3V pullup"
io8_spi_ft_ls_pd_3v3  "IO8_FT SPI low speed @ 3.3V pulldown"
io8_spi_hslv_ft_hs_1v2  "IO8_FT SPI HSLV high speed @ 1.2V"
io8_spi_hslv_ft_hs_pu_1v2  "IO8_FT SPI HSLV high speed @ 1.2V pullup"
io8_spi_hslv_ft_hs_pd_1v2  "IO8_FT SPI HSLV high speed @ 1.2V pulldown"
io8_spi_hslv_ft_fs_1v2  "IO8_FT SPI HSLV fast speed @ 1.2V"
io8_spi_hslv_ft_fs_pu_1v2  "IO8_FT SPI HSLV fast speed @ 1.2V pullup"
io8_spi_hslv_ft_fs_pd_1v2  "IO8_FT SPI HSLV fast speed @ 1.2V pulldown"
io8_spi_hslv_ft_ms_1v2  "IO8_FT SPI HSLV med speed @ 1.2V"
io8_spi_hslv_ft_ms_pu_1v2  "IO8_FT SPI HSLV med speed @ 1.2V pullup"
io8_spi_hslv_ft_ms_pd_1v2  "IO8_FT SPI HSLV med speed @ 1.2V pulldown"
io8_spi_hslv_ft_ls_1v2  "IO8_FT SPI HSLV low speed @ 1.2V"
io8_spi_hslv_ft_ls_pu_1v2  "IO8_FT SPI HSLV low speed @ 1.2V pullup"
io8_spi_hslv_ft_ls_pd_1v2  "IO8_FT SPI HSLV low speed @ 1.2V pulldown"
io8_spi_hslv_ft_hs_1v8  "IO8_FT SPI HSLV high speed @ 1.8V"
io8_spi_hslv_ft_hs_pu_1v8  "IO8_FT SPI HSLV high speed @ 1.8V pullup"
io8_spi_hslv_ft_hs_pd_1v8  "IO8_FT SPI HSLV high speed @ 1.8V pulldown"
io8_spi_hslv_ft_fs_1v8  "IO8_FT SPI HSLV fast speed @ 1.8V"
io8_spi_hslv_ft_fs_pu_1v8  "IO8_FT SPI HSLV fast speed @ 1.8V pullup"
io8_spi_hslv_ft_fs_pd_1v8  "IO8_FT SPI HSLV fast speed @ 1.8V pulldown"
io8_spi_hslv_ft_ms_1v8  "IO8_FT SPI HSLV med speed @ 1.8V"
io8_spi_hslv_ft_ms_pu_1v8  "IO8_FT SPI HSLV med speed @ 1.8V pullup"
io8_spi_hslv_ft_ms_pd_1v8  "IO8_FT SPI HSLV med speed @ 1.8V pulldown"
io8_spi_hslv_ft_ls_1v8  "IO8_FT SPI HSLV low speed @ 1.8V"
io8_spi_hslv_ft_ls_pu_1v8  "IO8_FT SPI HSLV low speed @ 1.8V pullup"
io8_spi_hslv_ft_ls_pd_1v8  "IO8_FT SPI HSLV low speed @ 1.8V pulldown"
io8_spi_hslv_ft_hs_2v5  "IO8_FT SPI HSLV high speed @ 2.5V"
io8_spi_hslv_ft_hs_pu_2v5  "IO8_FT SPI HSLV high speed @ 2.5V pullup"
io8_spi_hslv_ft_hs_pd_2v5  "IO8_FT SPI HSLV high speed @ 2.5V pulldown"
io8_spi_hslv_ft_fs_2v5  "IO8_FT SPI HSLV fast speed @ 2.5V"
io8_spi_hslv_ft_fs_pu_2v5  "IO8_FT SPI HSLV fast speed @ 2.5V pullup"
io8_spi_hslv_ft_fs_pd_2v5  "IO8_FT SPI HSLV fast speed @ 2.5V pulldown"
io8_spi_hslv_ft_ms_2v5  "IO8_FT SPI HSLV med speed @ 2.5V"
io8_spi_hslv_ft_ms_pu_2v5  "IO8_FT SPI HSLV med speed @ 2.5V pullup"
io8_spi_hslv_ft_ms_pd_2v5  "IO8_FT SPI HSLV med speed @ 2.5V pulldown"
io8_spi_hslv_ft_ls_2v5  "IO8_FT SPI HSLV low speed @ 2.5V"
io8_spi_hslv_ft_ls_pu_2v5  "IO8_FT SPI HSLV low speed @ 2.5V pullup"
io8_spi_hslv_ft_ls_pd_2v5  "IO8_FT SPI HSLV low speed @ 2.5V pulldown"
[Define Package Model]  481-lqfp-20x20-144-ldo-230228
[Manufacturer]  Unknown
[OEM]  Unknown
[Description]  None
[Number Of Pins]  136
[Pin Numbers]
| Pin Num   Terminal Name
25 | NRST
34 | PA0
102 | PA10
103 | PA11
104 | PA12
105 | PA13
109 | PA14
110 | PA15
35 | PA1
36 | PA2
37 | PA3
40 | PA4
41 | PA5
42 | PA6
43 | PA7
100 | PA8
101 | PA9
46 | PB0
69 | PB10
73 | PB12
74 | PB13
75 | PB14
76 | PB15
47 | PB1
48 | PB2
133 | PB3
134 | PB4
135 | PB5
136 | PB6
137 | PB7
139 | PB8
140 | PB9
26 | PC0
111 | PC10
112 | PC11
113 | PC12
7 | PC13
8 | PC14-OSC32_IN
9 | PC15-OSC32_OUT
27 | PC1
28 | PC2
29 | PC3
44 | PC4
45 | PC5
96 | PC6
97 | PC7
98 | PC8
99 | PC9
114 | PD0
79 | PD10
80 | PD11
81 | PD12
82 | PD13
85 | PD14
86 | PD15
115 | PD1
116 | PD2
117 | PD3
118 | PD4
119 | PD5
122 | PD6
123 | PD7
77 | PD8
78 | PD9
141 | PE0
63 | PE10
64 | PE11
65 | PE12
66 | PE13
67 | PE14
68 | PE15
142 | PE1
1 | PE2
2 | PE3
3 | PE4
4 | PE5
5 | PE6
58 | PE7
59 | PE8
60 | PE9
10 | PF0
22 | PF10
49 | PF11
50 | PF12
53 | PF13
54 | PF14
55 | PF15
11 | PF1
12 | PF2
13 | PF3
14 | PF4
15 | PF5
18 | PF6
19 | PF7
20 | PF8
21 | PF9
56 | PG0
125 | PG10
126 | PG11
127 | PG12
128 | PG13
129 | PG14
132 | PG15
57 | PG1
87 | PG2
88 | PG3
89 | PG4
90 | PG5
91 | PG6
92 | PG7
93 | PG8
124 | PG9
23 | PH0-OSC_IN
24 | PH1-OSC_OUT
138 | PH3-BOOT0
6 | VBAT
72 | VDD
108 | VDD
144 | VDD
39 | VDD
17 | VDD
52 | VDD
62 | VDD
84 | VDD
121 | VDD
70 | VCAP
106 | VDDUSB
33 | VDDA
95 | VDDIO2
131 | VDDIO2
31 | VREFM
32 | VREFP
16 | VSS
30 | VSSA
94 | VSS
130 | VSS
|[Merged Pins]  16
|38  |  VSS
|51  |  VSS
|61  |  VSS
|71  |  VSS
|83  |  VSS
|107  |  VSS
|120  |  VSS
|143  |  VSS
[Model Data]
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[End Model Data]
[End Package Model]
| Models and submodels in the file (265): io8_100m_ft_hs_1v2 (I/O), io8_100m_ft_hs_pu_1v2 (I/O), io8_100m_ft_hs_pd_1v2 (I/O), io8_100m_ft_fs_1v2 (I/O), io8_100m_ft_fs_pu_1v2 (I/O), io8_100m_ft_fs_pd_1v2 (I/O), io8_100m_ft_ms_1v2 (I/O), io8_100m_ft_ms_pu_1v2 (I/O), io8_100m_ft_ms_pd_1v2 (I/O), io8_100m_ft_ls_1v2 (I/O), io8_100m_ft_ls_pu_1v2 (I/O), io8_100m_ft_ls_pd_1v2 (I/O), io8_100m_ft_hs_1v8 (I/O), io8_100m_ft_hs_pu_1v8 (I/O), io8_100m_ft_hs_pd_1v8 (I/O), io8_100m_ft_fs_1v8 (I/O), io8_100m_ft_fs_pu_1v8 (I/O), io8_100m_ft_fs_pd_1v8 (I/O), io8_100m_ft_ms_1v8 (I/O), io8_100m_ft_ms_pu_1v8 (I/O), io8_100m_ft_ms_pd_1v8 (I/O), io8_100m_ft_ls_1v8 (I/O), io8_100m_ft_ls_pu_1v8 (I/O), io8_100m_ft_ls_pd_1v8 (I/O), io8_100m_ft_hs_3v3 (I/O), io8_100m_ft_hs_pu_3v3 (I/O), io8_100m_ft_hs_pd_3v3 (I/O), io8_100m_ft_fs_3v3 (I/O), io8_100m_ft_fs_pu_3v3 (I/O), io8_100m_ft_fs_pd_3v3 (I/O), io8_100m_ft_ms_3v3 (I/O), io8_100m_ft_ms_pu_3v3 (I/O), io8_100m_ft_ms_pd_3v3 (I/O), io8_100m_ft_ls_3v3 (I/O), io8_100m_ft_ls_pu_3v3 (I/O), io8_100m_ft_ls_pd_3v3 (I/O), io8_100m_hslv_ft_hs_1v2 (I/O), io8_100m_hslv_ft_hs_pu_1v2 (I/O), io8_100m_hslv_ft_hs_pd_1v2 (I/O), io8_100m_hslv_ft_fs_1v2 (I/O), io8_100m_hslv_ft_fs_pu_1v2 (I/O), io8_100m_hslv_ft_fs_pd_1v2 (I/O), io8_100m_hslv_ft_ms_1v2 (I/O), io8_100m_hslv_ft_ms_pu_1v2 (I/O), io8_100m_hslv_ft_ms_pd_1v2 (I/O), io8_100m_hslv_ft_ls_1v2 (I/O), io8_100m_hslv_ft_ls_pu_1v2 (I/O), io8_100m_hslv_ft_ls_pd_1v2 (I/O), io8_100m_hslv_ft_hs_1v8 (I/O), io8_100m_hslv_ft_hs_pu_1v8 (I/O), io8_100m_hslv_ft_hs_pd_1v8 (I/O), io8_100m_hslv_ft_fs_1v8 (I/O), io8_100m_hslv_ft_fs_pu_1v8 (I/O), io8_100m_hslv_ft_fs_pd_1v8 (I/O), io8_100m_hslv_ft_ms_1v8 (I/O), io8_100m_hslv_ft_ms_pu_1v8 (I/O), io8_100m_hslv_ft_ms_pd_1v8 (I/O), io8_100m_hslv_ft_ls_1v8 (I/O), io8_100m_hslv_ft_ls_pu_1v8 (I/O), io8_100m_hslv_ft_ls_pd_1v8 (I/O), io8_100m_hslv_ft_hs_2v5 (I/O), io8_100m_hslv_ft_hs_pu_2v5 (I/O), io8_100m_hslv_ft_hs_pd_2v5 (I/O), io8_100m_hslv_ft_fs_2v5 (I/O), io8_100m_hslv_ft_fs_pu_2v5 (I/O), io8_100m_hslv_ft_fs_pd_2v5 (I/O), io8_100m_hslv_ft_ms_2v5 (I/O), io8_100m_hslv_ft_ms_pu_2v5 (I/O), io8_100m_hslv_ft_ms_pd_2v5 (I/O), io8_100m_hslv_ft_ls_2v5 (I/O), io8_100m_hslv_ft_ls_pu_2v5 (I/O), io8_100m_hslv_ft_ls_pd_2v5 (I/O), io8_100m_i2c_ft_1v2 (I/O_open_drain), io8_100m_i2c_ft_pu_1v2 (I/O_open_drain), io8_100m_i2c_ft_pd_1v2 (I/O_open_drain), io8_100m_i2c_ft_1v8 (I/O_open_drain), io8_100m_i2c_ft_pu_1v8 (I/O_open_drain), io8_100m_i2c_ft_pd_1v8 (I/O_open_drain), io8_100m_i2c_ft_3v3 (I/O_open_drain), io8_100m_i2c_ft_pu_3v3 (I/O_open_drain)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
